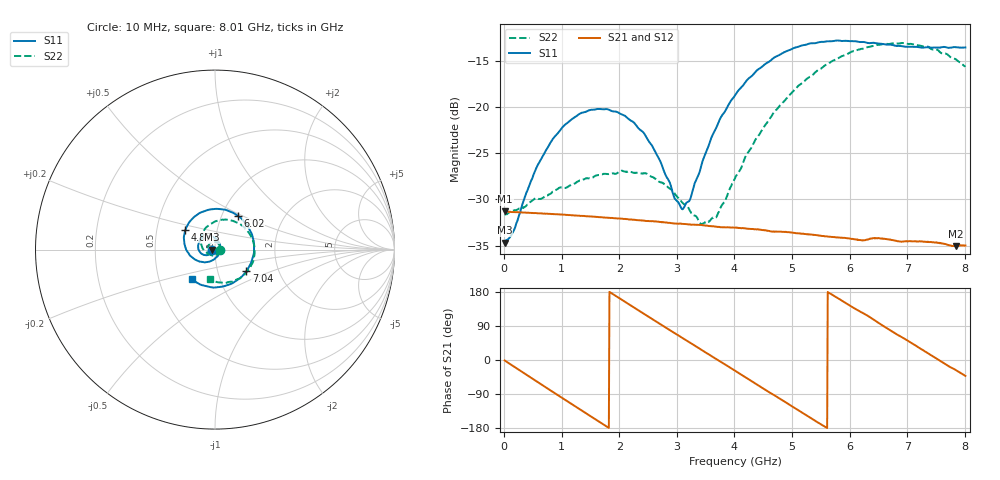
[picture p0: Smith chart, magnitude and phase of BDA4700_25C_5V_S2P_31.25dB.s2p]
!Agilent Technologies,E5071B,MY42404982,A.09.10
!Date: Mon Oct 20 13:42:22 2025
!Data & Calibration Information:
!Freq	S11:SOLT2(ON)	S21:SOLT2(ON)	S12:SOLT2(ON)	S22:SOLT2(ON)
# Hz S RI R 50
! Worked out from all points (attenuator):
!   801 points, 10 MHz to 8.01 GHz, reference 50 ohm
!   highest |S21| = -31.30 dB at 20 MHz (marker M1); lowest = -35.1 dB at 7.84 GHz (marker M2)
!   lowest |S11| = -34.7 dB at 10 MHz (marker M3), VSWR 1.04, Z = 48.2 - j0.0893 ohm
!   |S11| at or under -10 dB: start of sweep to end of sweep
!   |S22| runs from -32.7 to -13.1 dB; largest |S21 - S12| = 0.00027
!   S11 on the Smith chart (normalised r, x): 10 MHz: 0.96, -0.00; 4.87 GHz: 0.70, +0.16; 6.02 GHz: 1.19, +0.47; 7.04 GHz: 1.37, -0.35; 8.01 GHz: 0.73, -0.25
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1e7  -0.0184 -0.000926  0.0272 -0.000561  0.0272 -0.000604  0.0262 -0.000793
2e7  -0.0187 -0.00151  0.0272 -0.000991  0.0272 -0.00108  0.0261 -0.00112
1.6e8  -0.0191 -0.00911  0.0259 -0.00754  0.0259 -0.00756  0.0264 -0.00753
5.4e8  -0.0354 -0.0283  0.0157 -0.0216  0.0157 -0.0216  0.0157 -0.0278
7.7e8  -0.0529 -0.031  0.00616 -0.0257  0.00609 -0.0257  0.0011 -0.0335
1.35e9  -0.0931 0.00367  -0.0177 -0.0187  -0.0178 -0.0187  -0.036 -0.0178
2.09e9  -0.0533 0.0726  -0.0224 0.0107  -0.0224 0.0107  -0.0294 0.0338
2.68e9  0.0155 0.0509  -0.00322 0.0237  -0.0032 0.0237  0.0125 0.0375
2.97e9  0.029 0.0129  0.00794 0.022  0.00795 0.022  0.0255 0.0219
3.12e9  0.027 -0.00886  0.013 0.0193  0.013 0.0193  0.0281 0.00992
3.24e9  0.0202 -0.0251  0.0164 0.0162  0.0165 0.0162  0.027 0.0014
3.54e9  -0.0128 -0.0589  0.0219 0.00629  0.0218 0.00624  0.0131 -0.02
3.7e9  -0.0398 -0.0684  0.0225 0.00043  0.0225 0.000342  -0.000467 -0.0259
4.01e9  -0.0978 -0.0618  0.0196 -0.0105  0.0196 -0.0105  -0.032 -0.0257
4.87e9  -0.1647 0.111  -0.00715 -0.0198  -0.00706 -0.0199  -0.0743 0.0785
5.35e9  -0.0754 0.2084  -0.0185 -0.00849  -0.0185 -0.00853  -0.0153 0.1475
6.02e9  0.126 0.1892  -0.0153 0.0119  -0.0154 0.0119  0.1352 0.1451
6.68e9  0.2179 -0.00414  0.00308 0.0189  0.00312 0.0189  0.2196 0.000808
7.04e9  0.1745 -0.1208  0.0126 0.014  0.0127 0.0139  0.1979 -0.0955
7.46e9  0.0533 -0.2031  0.0183 0.00262  0.0183 0.00262  0.1112 -0.1723
7.84e9  -0.0795 -0.1951  0.0158 -0.00779  0.0158 -0.00788  0.0117 -0.1814
8.01e9  -0.1309 -0.1646  0.0132 -0.0119  0.0133 -0.0118  -0.0298 -0.1625
